PROGRAM PLCDBAutoLog
VAR
	fbPLCDBAutoLog					:FB_PLCDBAutoLog(sNetID:='' , tTimeout:=t#5s );
	bStartAutoLog					: BOOL;
END_VAR


IF bStartAutoLog THEN	
	fbPLCDBAutoLog.Start();
ELSE
	fbPLCDBAutoLog.Stop();
END_IF

END_PROGRAM
